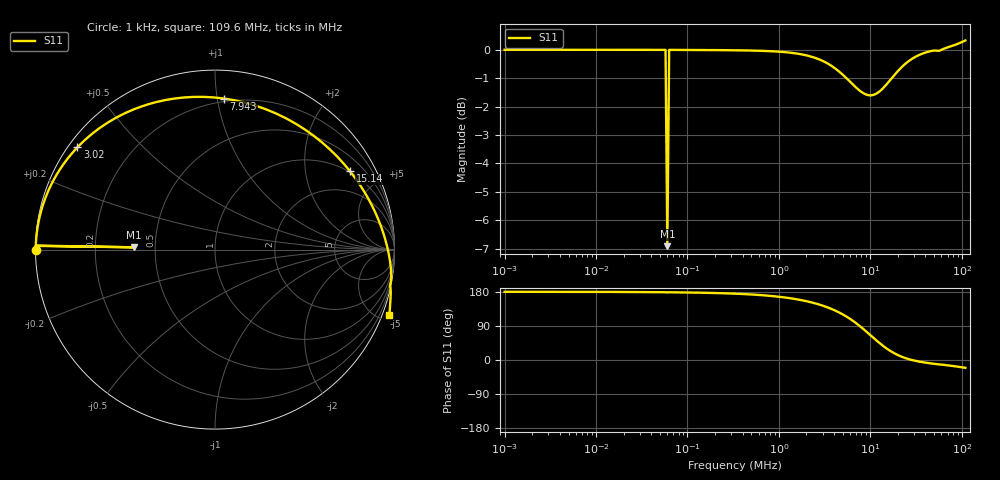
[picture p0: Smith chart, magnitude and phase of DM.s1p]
! EM Consulting and Software
! Touchstone file was created on 2026-03-05  19:00:34
# HZ S RI R 50.0000
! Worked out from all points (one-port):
!   253 points, 1 kHz to 109.6 MHz, reference 50 ohm
!   lowest |S11| = -6.9 dB at 60.26 kHz (marker M1), VSWR 2.65, Z = 18.9 + j0.608 ohm
!   |S11| at or under -10 dB: nowhere
!   S11 on the Smith chart (normalised r, x): 1 kHz: 0.00, +0.00; 3.02 MHz: 0.03, +0.33; 7.943 MHz: 0.18, +1.04; 15.14 MHz: 0.97, +3.47; 109.6 MHz: -0.57, -5.44
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1000  -0.9994 0.000424
4365.158  -0.9994 0.00181
18197.01  -0.9993 0.0074
57543.99  -0.9988 0.0206
60255.96  -0.4513 0.0128
63095.73  -0.9987 0.0222
79432.82  -0.9985 0.0267
331131.1  -0.9937 0.086
758577.6  -0.9784 0.1763
1445440  -0.936 0.3102
2187762  -0.8676 0.4414
3019952  -0.7667 0.5696
3630781  -0.6793 0.6495
4365158  -0.563 0.7281
5248075  -0.4125 0.7965
6025596  -0.2758 0.8334
6918310  -0.1202 0.8506
7943282  0.0495 0.8418
9120108  0.2253 0.8022
1.047129e7  0.3962 0.7312
1.258925e7  0.5977 0.596
1.513561e7  0.7523 0.4365
1.905461e7  0.8756 0.2431
2.630268e7  0.9539 0.0373
3.162278e7  0.9716 -0.0432
3.981072e7  0.9808 -0.1174
7.24436e7  0.9789 -0.2526
1.096478e8  0.9713 -0.3654
